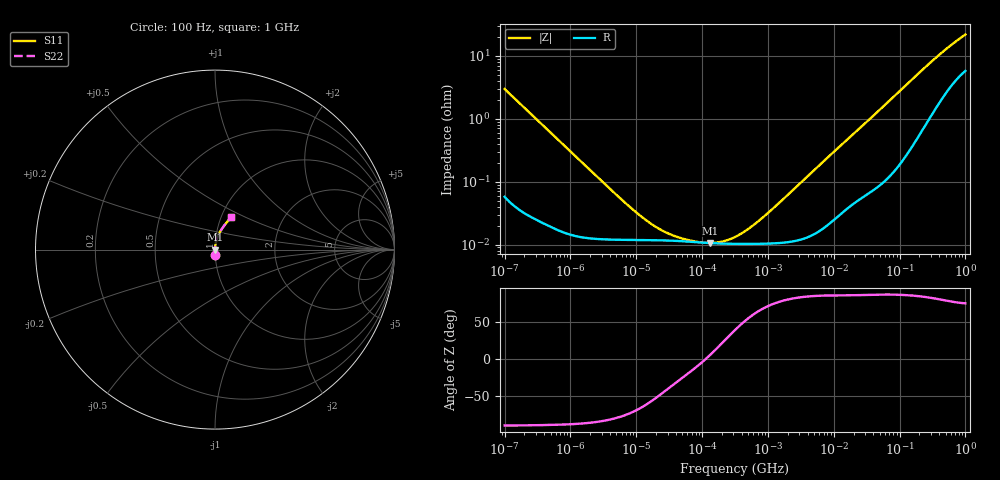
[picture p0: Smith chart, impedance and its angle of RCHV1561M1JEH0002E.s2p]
! RCHV1561M1JEH0002E  S-PARAMETER MODEL  (AEC-Q200 qualified)
! Model Generated by ELNA Corporation (http://www.ty-top.com)
! Version 1.0
! ELNA Control No.240229
! Copyright (c) 2024 ELNA CO.,LTD. All Rights Reserved.
! Products Name : CONDUCTIVE POLYMER HYBRID ALUMINUM ELECTROLYTIC CAPACITORS
! Characteristics :
!  Capacitance  :  560uF  ,  Rated voltage  :  6.3V
!  Operating Temp. Range  :  -55 to +105 degC  ,  Endurance  :  10000hr at 105 degC
!  Dimension D  :  8mm  ,  Dimension L  :  10mm
! Frequency Range : 100Hz - 1GHz
! External Node Assignments :
!  1  o---| |---o  2
# MHz S RI R 50
!Freq[MHz].  S11 Real  S11 Imag  S21 Real  S21 Imag  S12 Real  S12 Imag  S22 Real  S22 Imag
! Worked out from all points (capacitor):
!   401 points, 100 Hz to 1 GHz, reference 50 ohm
!   read as one part in series: C = 536 uF near 108 Hz
!   lowest |Z| = 10.6 mohm at 130.3 kHz (marker M1)
!   series resonance near 113.2 kHz, so ESL is about 3.7 nH
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0.0001  0.00145 -0.0296  0.9985 0.0296  0.9985 0.0296  0.00145 -0.0296
0.000113  0.00119 -0.0263  0.9988 0.0263  0.9988 0.0263  0.00119 -0.0263
0.001488  0.000135 -0.00203  0.9999 0.00203  0.9999 0.00203  0.000135 -0.00203
0.004597  0.00012 -0.000658  0.9999 0.000658  0.9999 0.000658  0.00012 -0.000658
0.00876  0.000118 -0.000345  0.9999 0.000345  0.9999 0.000345  0.000118 -0.000345
0.014207  0.000118 -0.000212  0.9999 0.000212  0.9999 0.000212  0.000118 -0.000212
0.022131  0.000117 -0.000135  0.9999 0.000135  0.9999 0.000135  0.000117 -0.000135
0.033113  0.000115 -8.75e-05  0.9999 8.75e-05  0.9999 8.75e-05  0.000115 -8.75e-05
0.051582  0.000113 -5.08e-05  0.9999 5.08e-05  0.9999 5.08e-05  0.000113 -5.08e-05
0.083657  0.000109 -1.9e-05  0.9999 1.9e-05  0.9999 1.9e-05  0.000109 -1.9e-05
0.130317  0.000106 9.21e-06  0.9999 -9.21e-06  0.9999 -9.21e-06  0.000106 9.21e-06
0.203002  0.000104 4.14e-05  0.9999 -4.14e-05  0.9999 -4.14e-05  0.000104 4.14e-05
0.316228  0.000103 8.28e-05  0.9999 -8.28e-05  0.9999 -8.28e-05  0.000103 8.28e-05
0.492606  0.000102 0.000141  0.9999 -0.000141  0.9999 -0.000141  0.000102 0.000141
0.798914  0.000103 0.000237  0.9999 -0.000237  0.9999 -0.000237  0.000103 0.000237
1.522299  0.000106 0.000459  0.9999 -0.000459  0.9999 -0.000459  0.000106 0.000459
4.704354  0.000143 0.00142  0.9999 -0.00142  0.9999 -0.00142  0.000143 0.00142
69.9842  0.00157 0.0192  0.9984 -0.0192  0.9984 -0.0192  0.00157 0.0192
169.8244  0.00624 0.0455  0.9938 -0.0455  0.9938 -0.0455  0.00624 0.0455
365.1741  0.0235 0.0906  0.9765 -0.0906  0.9765 -0.0906  0.0235 0.0906
641.9482  0.0544 0.1379  0.9456 -0.1379  0.9456 -0.1379  0.0544 0.1379
1000  0.0904 0.181  0.9096 -0.181  0.9096 -0.181  0.0904 0.181
